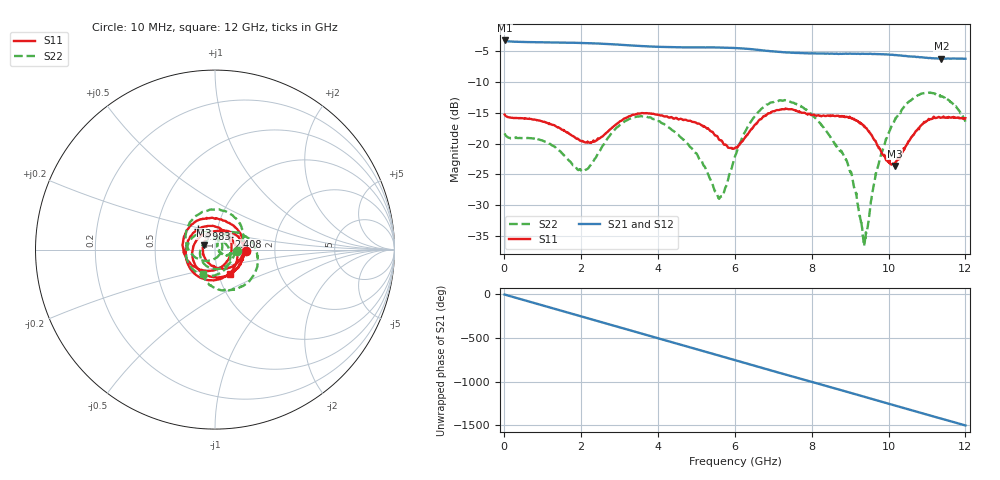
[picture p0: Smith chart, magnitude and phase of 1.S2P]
!Agilent Technologies,E5071C,MY46316741,A.11.02
!Date: Wed Sep 16 11:43:33 2020
!Data & Calibration Information:
!Freq	S11:SOLT2(ON)	S21:SOLT2(ON)	S12:SOLT2(ON)	S22:SOLT2(ON)
!PortZ  Port1:50+j0  Port2:50+j0
!Above PortZ is port z conversion or system Z0 setting when saving the data.
!When reading, reference impedance value at option line is always used.
# Hz S dB R 50
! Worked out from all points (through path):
!   1561 points, 10 MHz to 12 GHz, reference 50 ohm
!   highest |S21| = -3.25 dB at 10 MHz (marker M1); lowest = -6.2 dB at 11.38 GHz (marker M2)
!   group delay of S21, straight-line fit = 347 ps
!   lowest |S11| = -23.7 dB at 10.16 GHz (marker M3), VSWR 1.14, Z = 44.2 + j2.14 ohm
!   |S11| at or under -10 dB: start of sweep to end of sweep
!   |S22| runs from -36.7 to -11.7 dB; largest |S21 - S12| = 0.005
!   S11 on the Smith chart (normalised r, x): 10 MHz: 1.41, -0.02; 2.408 GHz: 1.15, +0.17; 4.983 GHz: 0.81, +0.19; 12 GHz: 1.14, -0.32
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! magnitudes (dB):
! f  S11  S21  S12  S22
! 10 MHz  -15.3  -3.2  -3.3  -18.4
! 1.124 GHz  -16.7  -3.6  -3.6  -19.9
! 2.016 GHz  -19.6  -3.7  -3.6  -24.5
! 2.408 GHz  -19.5  -3.7  -3.7  -22.0
! 3.177 GHz  -15.8  -4.0  -4.0  -16.3
! 4.007 GHz  -15.3  -4.3  -4.3  -16.4
! 4.983 GHz  -16.6  -4.4  -4.4  -21.5
! 5.613 GHz  -19.5  -4.4  -4.4  -28.8
! 6.005 GHz  -20.7  -4.5  -4.5  -22.1
! 6.389 GHz  -18.0  -4.6  -4.6  -16.8
! 6.866 GHz  -15.1  -4.9  -5.0  -13.6
! 7.404 GHz  -14.4  -5.2  -5.2  -13.1
! 8.011 GHz  -15.4  -5.3  -5.3  -15.3
! 8.91 GHz  -15.6  -5.4  -5.4  -22.8
! 9.079 GHz  -16.0  -5.4  -5.4  -26.3
! 9.379 GHz  -17.3  -5.4  -5.4  -36.1
! 9.679 GHz  -19.8  -5.5  -5.5  -24.6
! 10 GHz  -23.1  -5.5  -5.6  -18.3
! 10.16 GHz  -23.7  -5.6  -5.6  -16.3
! 10.8 GHz  -17.4  -6.0  -6.0  -12.1
! 11.38 GHz  -15.8  -6.2  -6.2  -12.3
! 12 GHz  -15.9  -6.2  -6.2  -16.5
